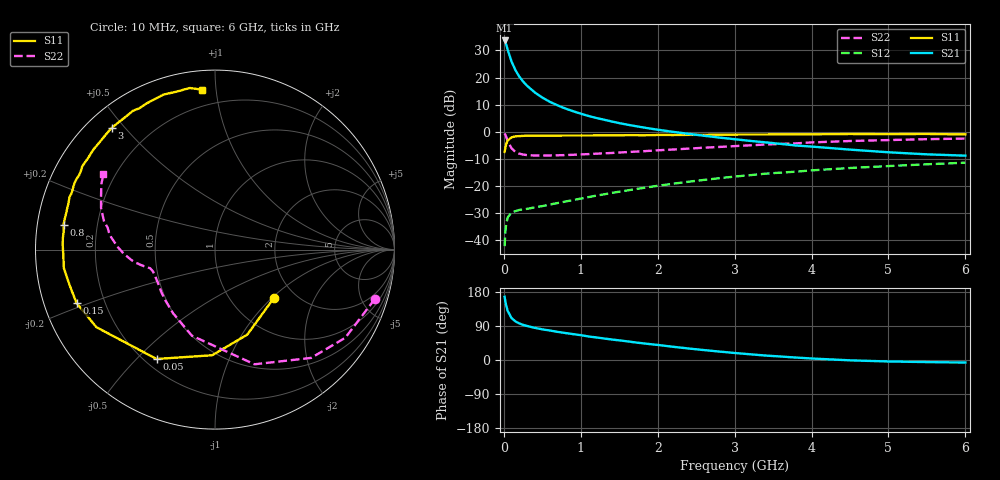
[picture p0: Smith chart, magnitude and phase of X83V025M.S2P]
! SIEMENS Small Signal Semiconductors
! BFP136W
! Si NPN RF Bipolar Junction Transistor in SOT343
! VCE = 3 V  IC = 25 mA
! Common Emitter S-Parameters:  September  1994
# GHz  S  MA  R  50
!  f  S11  S21  S12  S22
! GHz  MAG  ANG  MAG  ANG  MAG  ANG  MAG  ANG
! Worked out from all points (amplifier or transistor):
!   40 points, 10 MHz to 6 GHz, reference 50 ohm
!   highest |S21| = 33.7 dB at 10 MHz (marker M1)
!   |S21| within 3 dB of that: start of sweep to 45.63 MHz
!   unconditionally stable (mu >= 1): 823 MHz to 2.81 GHz
!   at 200 MHz: K = 0.38, MSG = 24.6 dB, |S12| = -28.8 dB
!   at 1.5 GHz: K = 1.14, MAG = 10.3 dB, |S12| = -22.1 dB
!   at 6 GHz: K = 0.98, MSG = 1.3 dB, |S12| = -11.4 dB
!   S11 on the Smith chart (normalised r, x): 10 MHz: 1.56, -1.03; 50 MHz: 0.25, -0.57; 150 MHz: 0.10, -0.18; 800 MHz: 0.08, +0.08; 3 GHz: 0.07, +0.46; 6 GHz: 0.10, +0.92
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0.01  0.4248 -39.7  48.18 166.9  0.0078 75.8  0.9322 -17.2
0.02  0.5067 -69.2  44.49 154.7  0.0144 68.4  0.8764 -34.1
0.03  0.5887 -91.5  40.81 144.6  0.0198 56.9  0.8068 -48.4
0.05  0.6909 -118.1  32.44 129.4  0.0264 44.2  0.6758 -71.0
0.1  0.7896 -146.8  19.71 110.8  0.0327 30.9  0.4968 -105.0
0.15  0.8266 -158.9  13.76 101.9  0.0345 27.5  0.4249 -123.3
0.2  0.8323 -165.3  10.43 96.6  0.0362 26.6  0.3953 -134.6
0.25  0.8406 -169.9  8.448 92.7  0.0373 26.6  0.3808 -142.0
0.3  0.8484 -173.1  7.085 89.8  0.0379 27.4  0.3713 -147.1
0.4  0.8457 -178.2  5.344 84.9  0.0405 30.9  0.3656 -153.7
0.5  0.8487 178.4  4.266 80.9  0.0427 33.8  0.3643 -157.7
0.6  0.8501 175.7  3.555 77.7  0.0457 36.7  0.3659 -160.1
0.7  0.8492 172.8  3.062 74.2  0.0487 39.7  0.3688 -161.6
0.8  0.855 170.6  2.68 71.2  0.0518 42.0  0.3724 -162.8
1.1  0.855 164.0  1.956 62.1  0.0625 47.1  0.3882 -165.2
1.5  0.8611 157.0  1.444 51.8  0.0786 51.4  0.4142 -167.6
2.2  0.8718 144.4  0.996 34.9  0.1104 52.3  0.471 -173.1
3  0.8892 130.4  0.73 18.5  0.1495 48.2  0.5449 178.2
3.2  0.8899 127.0  0.68 15.1  0.1587 46.9  0.5623 175.7
4.5  0.9101 108.4  0.469 -0.9  0.2152 35.6  0.6761 159.9
5.5  0.9114 98.9  0.384 -5.5  0.2518 27.3  0.7307 150.1
6  0.8941 94.6  0.363 -6.7  0.2695 22.8  0.7498 146.0
